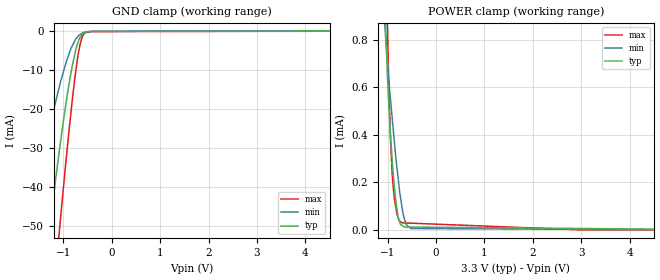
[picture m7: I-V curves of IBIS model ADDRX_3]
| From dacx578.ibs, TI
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|   ADDRX Model 3.3V MODEL
[Model] ADDRX_3
Model_type   Input
Vinl = 0.99
Vinh = 2.31
|   typ   min   max
|   (Nom PVT)   (Fast PVT)  (Slow PVT)
C_comp   3.2881350e-12   2.7087850e-12   3.8871290e-12
|Where nom PVT is Nom process, 3.3V, 27C
|Fast PVT is Strong Process, 3.6V, -40C
|Slow PVT is Weak Process,   3.0V, 125C
[Voltage Range]   3.3   3   3.6
[Temperature Range]   27   125   -40
|Junction temperatures are used for [Temperature Range]
[Power Clamp Reference]   3.3   3   3.6
[GND Clamp Reference]   0   0   0
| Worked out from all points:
|   GND clamp passes 1 mA (typ) near -0.63 V on its own axis
|   POWER clamp passes 1 mA (typ) near -1.06 V on its own axis
[GND Clamp]
|   Voltage   I(typ)   I(min)   I(max)
-3.3V     -294.8mA   -189.1mA   -371.7mA
-1.702V   -97.13mA   -52.41mA   -139.1mA
-1.309V   -53.06mA   -26.38mA   -82.53mA
-1.205V   -42.27mA   -20.5mA    -67.92mA
-1.095V   -31.49mA   -14.78mA   -52.69mA
-1.055V   -27.91mA   -12.79mA   -47.32mA
-901.2mV  -14.78mA   -6.412mA   -27.49mA
-760.2mV  -5.603mA   -2.335mA   -11.57mA
-663.9mV  -1.747mA   -921.6uA   -3.756mA
-609.3mV  -757.1uA   -495uA     -1.402mA
-420mV    -77.21uA   -92.29uA   -123.1uA
6.59V     0A         0A         0A
[POWER Clamp]
|   Voltage   I(typ)   I(min)   I(max)
-3.3V     26.61mA    20.54mA    32.86mA
-1.054V   939.2uA    845uA      1.333mA
-1.041V   853.9uA    804.3uA    1.204mA
-1.003V   636.1uA    702.3uA    829.5uA
-972.8mV  508.7uA    624.8uA    576.8uA
-943.2mV  404.8uA    553.1uA    389.1uA
-911.3mV  305.5uA    481.3uA    251.5uA
-888.9mV  242.7uA    431uA      187.6uA
-787.1mV  57.68uA    223.1uA    53.51uA
-658.1mV  12.4uA     50uA       29.73uA
-522.1mV  12.17uA    5.78uA     28.63uA
6.59V     0A         0A         0A
